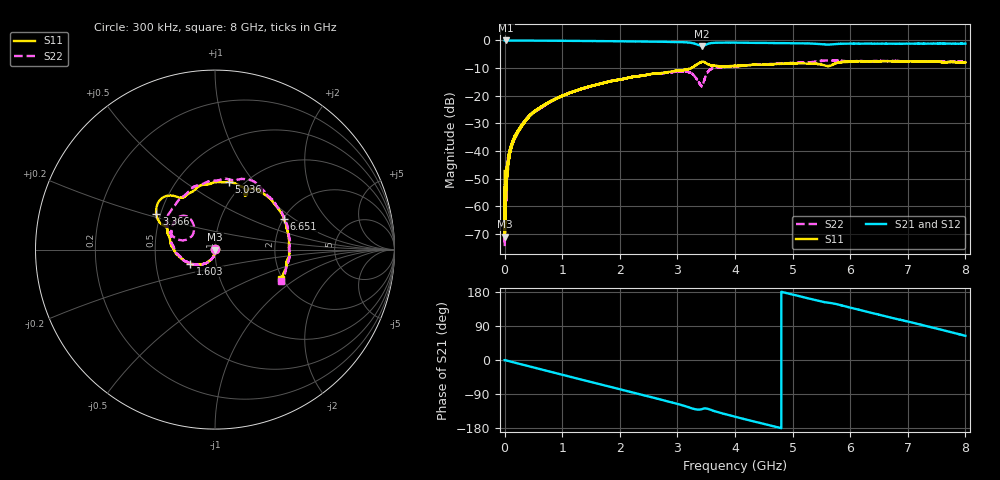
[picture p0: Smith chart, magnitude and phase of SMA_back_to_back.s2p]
#  HZ  S  DB  R  50.00
! Rohde & Schwarz ZVA/B
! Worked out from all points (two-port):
!   30000 points, 300 kHz to 8 GHz, reference 50 ohm
!   highest |S21| = 0.01 dB at 23.77 MHz (marker M1); lowest = -2.0 dB at 3.427 GHz (marker M2)
!   |S21| within 3 dB of the highest: start of sweep to end of sweep
!   lowest |S11| = -71.0 dB at 4.567 MHz (marker M3), VSWR 1.00, Z = 50 + j0.0281 ohm
!   |S11| at or under -10 dB: start of sweep to 3.239 GHz; 3.239276 GHz to 3.240624 GHz (1.348 MHz wide, 0.0416 % of centre)
!   |S22| runs from -74.5 to -7.2 dB; largest |S21 - S12| = 0.006
!   S11 on the Smith chart (normalised r, x): 300 kHz: 1.00, +0.01; 1.603 GHz: 0.75, -0.12; 3.366 GHz: 0.47, +0.22; 5.036 GHz: 0.86, +0.76; 6.651 GHz: 2.01, +0.84; 8 GHz: 1.97, -0.78
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300000  -47.27 115.2  0.00 -0.1  0.00 -0.1  -53.18 86.7
4566649  -71.03 90.1  0.01 -0.2  -0.00 -0.2  -60.78 -12.6
2.376657e7  -55.22 -95.3  0.01 -0.9  -0.01 -1.0  -53.13 -73.9
4.05665e7  -47.41 -85.1  -0.01 -1.6  -0.01 -1.6  -46.75 -89.5
7.203303e7  -42.88 -84.6  -0.01 -2.9  -0.02 -2.9  -42.94 -84.6
1.229662e8  -37.97 -88.6  -0.02 -4.9  -0.02 -4.9  -37.37 -89.0
3.677651e8  -28.94 -102.2  -0.04 -14.4  -0.05 -14.4  -28.97 -100.6
7.605635e8  -22.53 -118.7  -0.08 -29.6  -0.09 -29.5  -22.58 -117.2
1.333628e9  -17.49 -140.6  -0.17 -51.7  -0.17 -51.6  -17.62 -140.7
1.603493e9  -15.98 -150.6  -0.22 -62.0  -0.22 -61.9  -15.99 -152.4
2.666956e9  -11.93 169.4  -0.45 -102.7  -0.45 -102.5  -11.95 165.5
3.182687e9  -10.43 155.2  -0.72 -124.1  -0.70 -123.9  -11.37 137.6
3.366419e9  -8.33 148.6  -1.61 -131.0  -1.58 -130.8  -14.94 131.3
3.427486e9  -7.70 140.0  -1.95 -129.5  -1.93 -129.5  -16.39 151.4
3.592018e9  -9.00 124.8  -0.93 -132.2  -0.95 -132.0  -10.24 150.7
4.000283e9  -9.23 114.5  -0.78 -149.6  -0.77 -149.6  -9.30 124.6
5.036279e9  -8.28 78.2  -1.03 171.4  -1.03 171.5  -8.02 82.9
5.333611e9  -8.38 66.1  -1.12 160.2  -1.12 160.1  -7.82 72.8
6.650939e9  -7.53 24.1  -1.16 114.0  -1.15 113.9  -7.47 22.9
6.666939e9  -7.54 23.5  -1.16 113.3  -1.16 113.3  -7.46 22.4
7.324536e9  -7.70 0.8  -1.13 89.5  -1.15 89.2  -7.65 -1.4
8e9  -7.87 -24.1  -1.14 63.7  -1.16 63.9  -7.82 -26.2
